FUNCTION F_Crc4Legacy : BYTE
VAR_INPUT
END_VAR
VAR_IN_OUT
	aData			: ARRAY[*] OF USINT;
END_VAR
VAR
	nLowBoundData	: DINT;			// lower index
	nUpBoundData	: DINT;			// upper index
	nIdxCntData		: DINT;			// number elements
	
	aCrc4Table 		: ARRAY[0..255] OF BYTE:=[	0, 1, 2, 3, 4, 5, 6, 7, 8, 9, 10, 11, 12, 13, 14, 15,
												13, 12, 15, 14, 9, 8, 11, 10, 5, 4, 7, 6, 1, 0, 3, 2,
												7, 6, 5, 4, 3, 2, 1, 0, 15, 14, 13, 12, 11, 10, 9, 8,
												10, 11, 8, 9, 14, 15, 12, 13, 2, 3, 0, 1, 6, 7, 4, 5,
												14, 15, 12, 13, 10, 11, 8, 9, 6, 7, 4, 5, 2, 3, 0, 1,
												3, 2, 1, 0, 7, 6, 5, 4, 11, 10, 9, 8, 15, 14, 13, 12,
												9, 8, 11, 10, 13, 12, 15, 14, 1, 0, 3, 2, 5, 4, 7, 6,
												4, 5, 6, 7, 0, 1, 2, 3, 12, 13, 14, 15, 8, 9, 10, 11,
												1, 0, 3, 2, 5, 4, 7, 6, 9, 8, 11, 10, 13, 12, 15, 14,
												12, 13, 14, 15, 8, 9, 10, 11, 4, 5, 6, 7, 0, 1, 2, 3,
												6, 7, 4, 5, 2, 3, 0, 1, 14, 15, 12, 13, 10, 11, 8, 9,
												11, 10, 9, 8, 15, 14, 13, 12, 3, 2, 1, 0, 7, 6, 5, 4,
												15, 14, 13, 12, 11, 10, 9, 8, 7, 6, 5, 4, 3, 2, 1, 0,
												2, 3, 0, 1, 6, 7, 4, 5, 10, 11, 8, 9, 14, 15, 12, 13,
												8, 9, 10, 11, 12, 13, 14, 15, 0, 1, 2, 3, 4, 5, 6, 7,
												5, 4, 7, 6, 1, 0, 3, 2, 13, 12, 15, 14, 9, 8, 11, 10
												];		// CRC lookup table
	nIdx			: DINT;
	nRetBuff		: BYTE;
	temp			: BYTE;
END_VAR

// check if input array is not there
IF aData <> 0 THEN
	// get array dimensions 
	nLowBoundData := LOWER_BOUND(aData, 1);
	nUpBoundData := UPPER_BOUND(aData, 1);
	IF nLowBoundData = nUpBoundData THEN
		nIdxCntData := 1;
	ELSE
		nIdxCntData := nUpBoundData - nLowBoundData + 1;	
	END_IF


	nRetBuff:=5;
	
	FOR nIdx := nLowBoundData TO nUpBoundData DO
		temp := aData[nIdx] + (nRetBuff * 16);
		nRetBuff := aCrc4Table[temp];
	END_FOR
END_IF

 F_Crc4Legacy := nRetBuff;

END_FUNCTION
